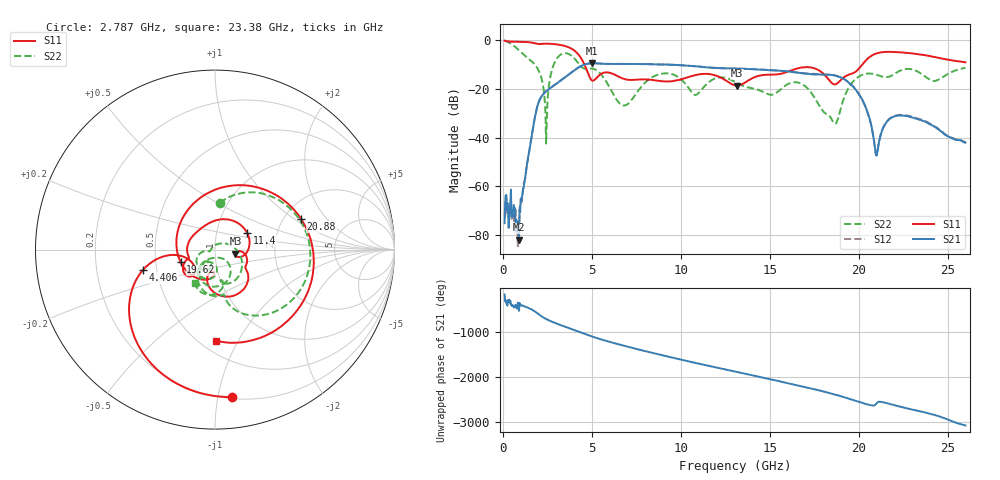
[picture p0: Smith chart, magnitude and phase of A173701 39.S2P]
!  2-Port S-parameters saved by WinCal
! VAR MeasName=S-Parameters (CALIBRATED_DATA) read from VNA (N5245A)
! VAR MeasDate=2017-6-7 10:31:00
! VAR NAME=A173701 39
! VAR FILENAME=A173701 39.S2P
! VAR DATE=2017-6-7 10:31:00
! VAR PHYS_PORTS=1,2
# Hz S DB R 50
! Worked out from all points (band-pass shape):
!   801 points, 100 MHz to 26 GHz, reference 50 ohm
!   highest |S21| = -9.56 dB at 5.021 GHz (marker M1); lowest = -81.9 dB at 909.4 MHz (marker M2)
!   |S21| within 3 dB of the highest: 4.002 GHz to 15.38 GHz (11.38 GHz wide, 117 % of centre); 15.38623 GHz to 15.43001 GHz (43.79 MHz wide, 0.284 % of centre)
!   lowest |S11| = -18.7 dB at 13.18 GHz (marker M3), VSWR 1.26, Z = 62.7 - j2.82 ohm
!   |S11| at or under -10 dB: 4.58 GHz to 20.22 GHz (15.64 GHz wide, 126 % of centre)
!   |S22| runs from -42.5 to -0.2 dB; largest |S21 - S12| = 0.0052
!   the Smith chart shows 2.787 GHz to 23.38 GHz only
!   S11 on the Smith chart (normalised r, x): 2.787 GHz: 0.21, -1.10; 4.406 GHz: 0.42, -0.12; 11.4 GHz: 1.41, +0.27; 19.62 GHz: 0.67, -0.10; 20.88 GHz: 2.47, +1.14; 23.38 GHz: 0.59, -0.82
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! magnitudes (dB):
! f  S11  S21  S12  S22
! 100 MHz  -0.3  -75.1  -70.6  -0.2
! 909.4 MHz  -0.8  -81.9  -83.1  -4.2
! 1.848 GHz  -1.5  -30.0  -30.0  -10.6
! 2.431 GHz  -1.6  -21.1  -21.1  -42.5
! 2.787 GHz  -1.7  -19.1  -19.1  -11.7
! 3.467 GHz  -2.4  -15.5  -15.4  -5.5
! 4.406 GHz  -7.6  -10.7  -10.7  -11.0
! 4.438 GHz  -8.0  -10.5  -10.5  -11.2
! 5.021 GHz  -16.7  -9.6  -9.6  -11.7
! 6.802 GHz  -16.0  -9.8  -9.8  -26.9
! 8.744 GHz  -16.7  -10.0  -10.0  -14.2
! 11.4 GHz  -13.9  -11.2  -11.2  -18.5
! 13.05 GHz  -18.6  -11.7  -11.7  -17.2
! 13.18 GHz  -18.7  -11.8  -11.8  -17.7
! 17.39 GHz  -11.4  -14.1  -13.9  -22.2
! 18.68 GHz  -18.2  -14.6  -14.6  -34.4
! 19.62 GHz  -13.8  -18.6  -18.6  -17.6
! 20.4 GHz  -8.5  -27.6  -27.8  -13.9
! 20.88 GHz  -5.9  -42.5  -42.4  -14.0
! 21.69 GHz  -4.9  -32.6  -32.5  -15.1
! 23.38 GHz  -5.9  -32.6  -32.4  -13.2
! 26 GHz  -9.2  -42.1  -42.2  -11.5
